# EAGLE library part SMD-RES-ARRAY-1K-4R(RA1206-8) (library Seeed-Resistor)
301030012
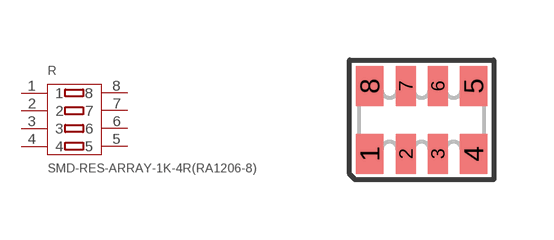
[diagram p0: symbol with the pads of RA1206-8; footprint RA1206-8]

Designator prefix R

## SMD-RES-ARRAY-1K-4R(RA1206-8) (MPN: Chip-Array-Series-1%; VALUE: 1K)  [RA1206-8]
1  1
2  2
3  3
4  4
5  5
6  6
7  7
8  8

## Footprint RA1206-8 (pad centres in mm)
BOURNS Chip Resistor Array Source: RS Component / BUORNS
smd 0.7 x 1: 1 -1.3,-0.85; 4 1.3,-0.85; 5 1.3,0.85; 8 -1.3,0.85
smd 0.5 x 1: 2 -0.4,-0.85; 3 0.4,-0.85; 6 0.4,0.85; 7 -0.4,0.85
